| Texas Instruments Incorporated
| TUSB9261 TUSB 3.0 to SATA Bridge
| Marketing part#   Voltage Range   Package-type   Temperature
| TUSB9261PAP   2.97V - 3.465V   64-Pin TQFP   -40 to 105 C
| TUSB9261PVP   2.97V - 3.465V   64-Pin TQFP   -40 to 105 C
[IBIS Ver]   4.0
[File name]   tusb9261.ibs
[File Rev]   1.0
[Date]   12/17/2010
[Source]   Model built from TISPICE simulations at:
   Texas Instruments Incorporated.
   Analog-eLab, HPA
   12500 TI Blvd
   Dallas, TX -75243
   For Support e-mail: elab_scm_ibis@list.ti.com
[Notes]   Rev 1.0: 12/17/2010
   - Model based on tusb1310.ibs v1.1 IBIS model.
   - Model generated from simulations in TISPICED
   - For USB2.0, models are included for HS, FS and LS modes
   - For USB3.0, models are included for SATA1, SATA2 and No-De-Emphasis
   modes
   - USB2 and USB3  models are matched to TISPICE.
   - Added model for DeEmphasis mode
   - Please use [Package Model] for system analysis
   - C_comp although listed in numerical order of value are obtained from varying
   PVT conditions. For PVT conditions for each specific value refer the buffer
   description under respective [Model]. IBIS model user is responsible for using
   appropriate C_comp to simulate for Signal Integrity
   Where for TUSB1310,
   Nom PVT:  Nominal process, Typ Temperature, Typ Voltage
   Slow PVT: Weak process, Max Temperature, Min Voltage
   Fast PVT: Strong process, Min Temperature, Max Voltage
   - ignore warning are related to usb3_WODE, please do not correct this error
   as IBIS parser does not correct IV-VT mismatch with single set of V-T
   waveforms.
   - non-monotonic arnings related to usb2_LS_RC and usb2_LS_R buffers are
   as they are seen in TISPICE simualations
   - [Driver Schedule] is interpreted differently by each system level simulator
   differently, if usual setup with it does not give appropriate results, please
   tie the MAIN and BOOST buffers as per buffer timing description under
   [Driver Schedule] keyword. For example, using HSPICE, refer DE_hspice.sp
   - To test USB2 IBIS models using HSPICE look for spice set up files
   inside the TUSB1310 Correlation report
   - Both PVP and PAP packages have same parasitics
   - Digital models are from standard ASIC SR60 IBIS library for TUSB9261
[Disclaimer] This product is designed as an aid for customers of Texas Instruments.
   No warranties, either expressed or implied, with respect to this third
   party software (if any) or with respect to its fitness for any
   particular purpose is claimed by Texas Instruments or the author. The
   software (if any) is provided solely on an "as is" basis. The entire
   risk as to its quality and performance is with the customer
[Copyright]   (C)Copyright 2010 Texas Instruments Incorporated.
   All rights reserved.
|   TUSB9261 PAP 64-pin TQFP with thermal pad
[Component]   TUSB9261PAP
[Manufacturer]  Texas Instruments Incorporated
[Package]   |65-pin PAP TQFP
|   typ   min   max
R_pkg   0.211135   0.01351   0.24747
L_pkg   2.91049nH   1.34206nH   3.55002nH
C_pkg   0.62782pF   0.45374pF   0.68688pF
[PIN]  Signal_name   Model_name   R_pin   L_pin   C_pin
1   VDD   POWER   0.13086   3.225576nH   0.70225pF
2   PWM0   BC3340DSHYPBFZP18PD  0.23767   3.369912nH   0.67131pF
3   PWM1   BC3340DSHYPBFZP18PD  0.22511   3.211136nH   0.65435pF
4   GRSTZ   IC33SHYPBFZP18PU   0.21557   3.084096nH   0.63183pF
5   UART_RX_GPIO8  BC3340DSHYPBFZP18PU  0.21063   3.003016nH   0.62696pF
6   UART_TX_GPIO9  BC3340DSHYPBFZP18PU  0.20875   2.955072nH   0.62244pF
7   VDD33   POWER   0.10961   2.607272nH   0.64774pF
8   GPIO0   BC3340DSHYPBFZP18PD  0.20588   2.88772nH   0.58903pF
9   GPIO1   BC3340DSHYPBFZP18PD  0.20559   2.88536nH   0.5925pF
10   GPIO2   BC3340DSHYPBFZP18PD  0.20518   2.898064nH   0.61553pF
11   GPIO3   BC3340DSHYPBFZP18PD  0.20774   2.947056nH   0.60753pF
12   VDD   POWER   0.11187   2.699616nH   0.66867pF
13   GPIO4   BC3340DSHYPBFZP18PD  0.21619   3.092752nH   0.64028pF
14   GPIO5   BC3340DSHYPBFZP18PD  0.2259   3.222312nH   0.66752pF
15   GPIO6   BC3340DSHYPBFZP18PD  0.23204   3.320784nH   0.68037pF
16   GPIO7   BC3340DSHYPBFZP18PD  0.24662   3.541544nH   0.62837pF
17   SPI_SCLK   BC3340DSHYPBFZP18PU  0.24747   3.550024nH   0.64185pF
18   SPI_DATA_IN   IC33SHYPBFZP18PU   0.23987   3.395592nH   0.68688pF
19   VDD   POWER   0.12307   2.9634nH   0.71297pF
20   SPI_DATA_OUT   BC3340DSHYPBFZP18PU  0.2236   3.164256nH   0.65587pF
21   SPI_CS0   BC3340DSHYPBFZP18PU  0.22022   3.097736nH   0.6409pF
22   SPI_CS1_GPIO10 BC3340DSHYPBFZP18PU  0.21452   3.013472nH   0.61593pF
23   SPI_CS2_GPIO11 BC3340DSHYPBFZP18PU  0.21142   2.959624nH   0.60709pF
24   VDD33   POWER   0.112   2.631416nH   0.65058pF
25   JTAG_TCK   IC33SHYPBFZP18PD   0.21142   2.94336nH   0.59887pF
26   JTAG_TDI   IC33SHYPBFZP18PU   0.21121   2.957824nH   0.62272pF
27   JTAG_TDO   BC3340DSHYPBFZP18PD  0.21414   3.009856nH   0.61076pF
28   JTAG_TMS   IC33SHYPBFZP18PU   0.21773   3.074424nH   0.62341pF
29   JTAG_TRSTZ   IC33SHYPBFZP18PD   0.22537   3.180992nH   0.65602pF
30   FREQSEL0   IC33SHYPBFZP18PU   0.22999   3.262152nH   0.66926pF
31   FREQSEL1   IC33SHYPBFZP18PU   0.24224   3.418064nH   0.67295pF
32   VDD   POWER   0.09526   3.587624nH   0.70248pF
33   VDD   POWER   0.26179   3.685304nH   0.65998pF
34   VDDA33   POWER   0.23867   3.383512nH   0.67901pF
35   USB_DM   usb2   0.2264   3.226896nH   0.65519pF
36   USB_DP   usb2   0.21671   3.097536nH   0.63419pF
37   NC   NC   0.01351   1.342056nH   0.47338pF
38   USB_R1   NC   0.2087   2.956272nH   0.60989pF
39   USB_R1RTN   NC   0.20571   2.903064nH   0.5999pF
40   VDDA33   POWER   0.2054   2.88348nH   0.59106pF
41   VDD   POWER   0.08086   2.864096nH   0.65481pF
42   USB_SSTX_N   usb3   0.20711   2.186388nH   0.60301pF
43   USB_SSTX_P   usb3   0.21108   2.232552nH   0.61344pF
44   NC   NC   0.21761   3.068664nH   0.62787pF
45   USB_SSRX_N   RXP_N   0.22603   2.386884nH   0.66154pF
46   USB_SSRX_P   RXP_N   0.23763   2.496954nH   0.6838pF
47   VDD   POWER   0.09682   3.705672nH   0.78409pF
48   VDDR33   POWER   0.27024   3.760504nH   0.65113pF
49   VDD   POWER   0.09565   3.189344nH   0.7401pF
50   USB_VBUS   NC   0.24038   3.394712nH   0.67398pF
51   VDD33   POWER   0.12314   2.989664nH   0.71237pF
52   XI   NC   0.22287   3.151136nH   0.64979pF
53   VSSOSC   GND   0.21544   3.046216nH   0.63062pF
54   XO   NC   0.2111   2.974672nH   0.63043pF
55   VDD   POWER   0.11418   2.729152nH   0.6819pF
56   SATA_TX_N   SATA   0.21102   2.19969nH   0.59907pF
57   SATA_TX_P   SATA   0.21296   2.2134nH   0.59744pF
58   NC   NC   0.21605   2.996784nH   0.61426pF
59   SATA_RX_N   RXP_N   0.22106   2.301492nH   0.64313pF
60   SATA_RX_P   RXP_N   0.22882   2.379558nH   0.64598pF
61   VDD   POWER   0.0925   3.52468nH   0.7389pF
62   VDDR33   POWER   0.25481   3.491112nH   0.67158pF
63   VDD   POWER   0.25401   3.523744nH   0.67646pF
64   NC   NC   0.01425   1.544184nH   0.45374pF
65   VSS   GND   0.0001   0.0001nH   0.0001pF|THERMAL PAD
|   TUSB9261 PVP 64-pin TQFP with thermal pad
[Component]   TUSB9261PVP
[Manufacturer]  Texas Instruments Incorporated
[Package]   |65-pin PVP TQFP
|   typ   min   max
R_pkg   0.211135   0.01351   0.24747
L_pkg   2.22301nH   0.82343nH   2.83923nH
C_pkg   0.626679pF   0.45374pF   0.68688pF
[PIN]  Signal_name   Model_name   R_pin   L_pin   C_pin
1   VDD   POWER   0.13086   2.466064nH   0.70225pF
2   PWM0   BC3340DSHYPBFZP18PD  0.23767   2.671448nH   0.67131pF
3   PWM1   BC3340DSHYPBFZP18PD  0.22511   2.515544nH   0.65435pF
4   GRSTZ   IC33SHYPBFZP18PU   0.21557   2.365448nH   0.63183pF
5   UART_RX_GPIO8  BC3340DSHYPBFZP18PU  0.21063   3.003016nH   0.62696pF
6   UART_TX_GPIO9  BC3340DSHYPBFZP18PU  0.20875   2.278152nH   0.62244pF
7   VDD33   POWER   0.10961   1.910424nH   0.64774pF
8   GPIO0   BC3340DSHYPBFZP18PD  0.20588   2.142112nH   0.58903pF
9   GPIO1   BC3340DSHYPBFZP18PD  0.20559   2.150664nH   0.5925pF
10   GPIO2   BC3340DSHYPBFZP18PD  0.20518   2.180696nH   0.61553pF
11   GPIO3   BC3340DSHYPBFZP18PD  0.20774   2.223272nH   0.60753pF
12   VDD   POWER   0.11187   1.988264nH   0.66867pF
13   GPIO4   BC3340DSHYPBFZP18PD  0.21619   2.37416nH   0.64028pF
14   GPIO5   BC3340DSHYPBFZP18PD  0.2259   2.526576nH   0.66752pF
15   GPIO6   BC3340DSHYPBFZP18PD  0.23204   2.624064nH   0.68037pF
16   GPIO7   BC3340DSHYPBFZP18PD  0.24662   2.837376nH   0.62837pF
17   SPI_SCLK   BC3340DSHYPBFZP18PU  0.24747   2.839232nH   0.64185pF
18   SPI_DATA_IN   IC33SHYPBFZP18PU   0.23987   2.697288nH   0.68688pF
19   VDD   POWER   0.12307   2.274824nH   0.71297pF
20   SPI_DATA_OUT   BC3340DSHYPBFZP18PU  0.2236   2.445128nH   0.65587pF
21   SPI_CS0   BC3340DSHYPBFZP18PU  0.22022   2.372392nH   0.6409pF
22   SPI_CS1_GPIO10 BC3340DSHYPBFZP18PU  0.21452   2.289296nH   0.61593pF
23   SPI_CS2_GPIO11 BC3340DSHYPBFZP18PU  0.21142   2.2416nH   0.60709pF
24   VDD33   POWER   0.112   1.90852nH   0.65058pF
25   JTAG_TCK   IC33SHYPBFZP18PD   0.21142   2.208344nH   0.59887pF
26   JTAG_TDI   IC33SHYPBFZP18PU   0.21121   2.239896nH   0.62272pF
27   JTAG_TDO   BC3340DSHYPBFZP18PD  0.21414   2.285672nH   0.61076pF
28   JTAG_TMS   IC33SHYPBFZP18PU   0.21773   2.348848nH   0.62341pF
29   JTAG_TRSTZ   IC33SHYPBFZP18PD   0.22537   2.46208nH   0.65602pF
30   FREQSEL0   IC33SHYPBFZP18PU   0.22999   2.566816nH   0.66926pF
31   FREQSEL1   IC33SHYPBFZP18PU   0.24224   2.721184nH   0.67295pF
32   VDD   POWER   0.09526   2.467272nH   0.70248pF
33   VDD   POWER   0.26179   2.976512nH   0.65998pF
34   VDDA33   POWER   0.23867   2.685288nH   0.67901pF
35   USB_DM   usb2   0.2264   2.531224nH   0.65519pF
36   USB_DP   usb2   0.21671   2.378968nH   0.63419pF
37   NC   NC   0.01351   0.823432nH   0.47338pF
38   USB_R1   NC   0.2087   2.232496nH   0.60989pF
39   USB_R1RTN   NC   0.20571   2.18544nH   0.5999pF
40   VDDA33   POWER   0.2054   2.137712nH   0.59106pF
41   VDD   POWER   0.08086   2.121728nH   0.65481pF
42   USB_SSTX_N   usb3   0.20711   1.648002nH   0.60301pF
43   USB_SSTX_P   usb3   0.21108   1.689534nH   0.61344pF
44   NC   NC   0.21761   2.343088nH   0.62787pF
45   USB_SSRX_N   RXP_N   0.22603   1.975452nH   0.66154pF
46   USB_SSRX_P   RXP_N   0.23763   1.975452nH   0.6838pF
47   VDD   POWER   0.09682   3.020784nH   0.78409pF
48   VDDR33   POWER   0.27024   3.058096nH   0.65113pF
49   VDD   POWER   0.09565   2.215056nH   0.7401pF
50   USB_VBUS   NC   0.24038   2.696408nH   0.67398pF
51   VDD33   POWER   0.12314   2.297232nH   0.71237pF
52   XI   NC   0.22287   2.432248nH   0.64979pF
53   VSSOSC   GND   0.21544   2.321352nH   0.63062pF
54   XO   NC   0.2111   2.251696nH   0.63043pF
55   VDD   POWER   0.11418   2.015832nH   0.6819pF
56   SATA_TX_N   SATA   0.21102   1.640724nH   0.59907pF
57   SATA_TX_P   SATA   0.21296   1.662558nH   0.59744pF
58   NC   NC   0.21605   2.279256nH   0.61426pF
59   SATA_RX_N   RXP_N   0.22106   1.758834nH   0.64313pF
60   SATA_RX_P   RXP_N   0.22882   1.835676nH   0.64598pF
61   VDD   POWER   0.0925   2.631208nH   0.7389pF
62   VDDR33   POWER   0.25481   2.795136nH   0.67158pF
63   VDD   POWER   0.25401   2.826544nH   0.67646pF
64   NC   NC   0.01425   0.983936nH   0.45374pF
65   VSS   GND   0.0001   0.0001nH   0.0001pF|THERMAL PAD
[Diff_pin]   inv_pin   vdiff   tdelay_typ   tdelay_min   tdelay_max
36   35   880mV   NA NA NA|USB_DP/DM
43   42   NA   NA NA NA| USB_SSTXP/N
46   45   2200mV   NA NA NA| USB_SSRXP/N
57   56   NA   NA NA NA| SATA_TXP/N
60   59   2200mV   NA NA NA| SATA_RXP/N
[Pin Mapping] pulldown_ref pullup_ref gnd_clamp_ref power_clamp_ref |ext_ref
1   NC   VDD11BUS
2   VSSBUS   VDD33BUS   VSSBUS   VDD33BUS
3   VSSBUS   VDD33BUS   VSSBUS   VDD33BUS
4   NC   NC   VSSBUS   VDD33BUS
5   VSSBUS   VDD33BUS   VSSBUS   VDD33BUS
6   VSSBUS   VDD33BUS   VSSBUS   VDD33BUS
7   NC   VDD33BUS
8   VSSBUS   VDD33BUS   VSSBUS   VDD33BUS
9   VSSBUS   VDD33BUS   VSSBUS   VDD33BUS
10   VSSBUS   VDD33BUS   VSSBUS   VDD33BUS
11   VSSBUS   VDD33BUS   VSSBUS   VDD33BUS
12   NC   VDD11BUS
13   VSSBUS   VDD33BUS   VSSBUS   VDD33BUS
14   VSSBUS   VDD33BUS   VSSBUS   VDD33BUS
15   VSSBUS   VDD33BUS   VSSBUS   VDD33BUS
16   VSSBUS   VDD33BUS   VSSBUS   VDD33BUS
17   VSSBUS   VDD33BUS   VSSBUS   VDD33BUS
18   NC   NC   VSSBUS   VDD33BUS
19   NC   VDD11BUS
20   VSSBUS   VDD33BUS   VSSBUS   VDD33BUS
21   VSSBUS   VDD33BUS   VSSBUS   VDD33BUS
22   VSSBUS   VDD33BUS   VSSBUS   VDD33BUS
23   VSSBUS   VDD33BUS   VSSBUS   VDD33BUS
24   NC   VDD33BUS
25   NC   NC   VSSBUS   VDD33BUS
26   NC   NC   VSSBUS   VDD33BUS
27   VSSBUS   VDD33BUS   VSSBUS   VDD33BUS
28   NC   NC   VSSBUS   VDD33BUS
29   NC   NC   VSSBUS   VDD33BUS
30   NC   NC   VSSBUS   VDD33BUS
31   NC   NC   VSSBUS   VDD33BUS
32   NC   VDD11BUS
33   NC   VDD11BUS
34   NC   VDDA33BUS
35   VSSBUS   VDD33BUS   VSSBUS   VDD33BUS
36   VSSBUS   VDD33BUS   VSSBUS   VDD33BUS
37   NC   NC
38   NC   NC
39   NC   NC
40   NC   VDDA33
41   NC   VDD11BUS
42   VSSBUS   VDD11BUS   VSSBUS   VDD11BUS
43   VSSBUS   VDD11BUS   VSSBUS   VDD11BUS
44   NC   NC
45   NC   NC   VSSBUS   VDD11BUS
46   NC   NC   VSSBUS   VDD11BUS
47   NC   VDD11BUS
48   NC   VDDR33BUS
49   NC   VDD11BUS
50   NC   NC
51   NC   VDD33BUS
52   NC   NC
53   VSSBUS   NC
54   NC   NC
55   NC   VDD11BUS
56   VSSBUS   VDD11BUS   VSSBUS   VDD11BUS
57   VSSBUS   VDD11BUS   VSSBUS   VDD11BUS
58   NC   NC
59   NC   NC   VSSBUS   VDD11BUS
60   NC   NC   VSSBUS   VDD11BUS
61   NC   VDD11BUS
62   NC   VDDR33BUS
63   NC   VDD11BUS
64   NC   NC
65   VSSBUS   NC
[Model Selector] usb2
usb2_HS_R   USB 2.0 High Speed mode, for DP/DM pin 240MHz
usb2_HS_RC   USB 2.0 High Speed mode, for DP/DM pin 240MHz, with Cfixture
usb2_FS_R   USB 2.0 Fast Speed mode, for DP/DM pin 6MHz
usb2_FS_RC   USB 2.0 Fast Speed mode, for DP/DM pin 6MHz, with Cfixture
usb2_LS_RC   USB 2.0 Low  Speed mode, for DP/DM pin 750kHz, with Cfixture
usb2_LS_R   USB 2.0 Low  Speed mode, for DP/DM pin 750kHz
[Model Selector] usb3
usb3_DE   USB 3.0 De-Emphasis mode, best at 1.25GHz
usb3_WODE   USB 3.0 No De-Emphasis mode, for SSTXP/N 2.5GHz
usb3_SATA1   USB 3.0 SATA1 mode, for SSTXP/N 750MHz
usb3_SATA2   USB 3.0 SATA2 mode, for SSTXP/N 1.5GHz
[Model Selector] SATA
usb3_SATA1   USB 3.0 SATA1 mode, for SSTXP/N 750MHz
usb3_SATA2   USB 3.0 SATA2 mode, for SSTXP/N 1.5GHz
[Model Selector] BC3340DSHYPBFZP18
HYPBFZP18_PI_5P_3P3 BUFFER WITHOUT PULLUP/PULLDOWN & 5% VDDS TOLERANCE
HYPBFZP18_PI_10P_3P3 BUFFER WITHOUT PULLUP/PULLDOWN & 10% VDDS TOLERANCE
[Model Selector] BC3340DSHYPBFZP18PU
FZP18_PU_PI_5P_3P3 BUFFER WITH WEAK PULLUP & 5% VDDS TOLERANCE
FZP18_PU_PI_10P_3P3 BUFFER WITH WEAK PULLUP & 10% VDDS TOLERANCE
[Model Selector] BC3340DSHYPBFZP18PD
FZP18_PD_PI_5P_3P3 BUFFER WITH WEAK PULLDOWN & 5% VDDS TOLERANCE
FZP18_PD_PI_10P_3P3 BUFFER WITH WEAK PULLDOWN & 10% VDDS TOLERANCE
[Model Selector] IC33SHYPBFZP18
C33SHYPBFZP18_10P BUFFER WITHOUT PULLUP/PULLDOWN & 10% VDDS TOLERANCE
C33SHYPBFZP18_5P  BUFFER WITHOUT PULLUP/PULLDOWN & 5% VDDS TOLERANCE
[Model Selector] IC33SHYPBFZP18PD
YPBFZP18_PD_5P BUFFER with WEAK PULLDOWN & 5% VDDS TOLERANCE
YPBFZP18_PD_10P BUFFER with WEAK PULLDOWN & 5% VDDS TOLERANCE
[Model Selector] IC33SHYPBFZP18PU
PBFZP18_PU_5P BUFFER with WEAK PULLUP & 5% VDDS TOLERANCE
PBFZP18_PU_10P BUFFER with WEAK PULLUP & 10% VDDS TOLERANCE
|USB 3.0 De-Emphasis mode, for SSTXP/SSTXN pins 2.5Gbps(1.25GHz to De-Emphasis)
[Model]   usb3_DE
Model_type   Output
Vmeas = 1.1
Vref = 1.1
Rref = 50
|   typ   min   max
|   (TYP PVT)   (Fast PVT) (Slow PVT)
C_comp   0pF   0pF   0pF
[Driver Schedule]
| Model_name   Rise_on_dly Rise_off_dly Fall_on_dly Fall_off_dly
usb3_de_MAIN   0.0nS   0.4ns   0   0.4ns
usb3_de_BOOST   0.0nS   0.2nS   0   0.2nS
[Voltage Range]   1.1   0.99   1.155
[Temperature Range]   27   105   -40
[Pullup Reference]   1.1   0.99   1.155
[Pulldown Reference]   0   0   0
[Power Clamp Reference]   1.1   0.99   1.155
[GND Clamp Reference]   0   0   0
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[Ramp]
R_load = 50
|   typ   min   max
dV/dt_r   0.972315/1.549e-011   0.988218/1.8606e-011   0.957162/1.40763e-011
dV/dt_f   0.972312/7.7916e-012   0.988183/1.21282e-011  0.957081/6.00194e-012
| Models and submodels in the file (25): RXP_N (Input), usb2_FS_R (I/O), usb2_FS_RC (I/O), usb2_HS_R (I/O), usb2_HS_RC (I/O), usb2_LS_R (I/O), usb2_LS_RC (I/O), usb3_WODE (Output), usb3_SATA1 (Output), usb3_SATA2 (Output), usb3_DE (Output), usb3_de_MAIN (Output), usb3_de_BOOST (Open_drain), HYPBFZP18_PI_5P_3P3 (I/O), HYPBFZP18_PI_10P_3P3 (I/O), FZP18_PU_PI_5P_3P3 (I/O), FZP18_PU_PI_10P_3P3 (I/O), FZP18_PD_PI_5P_3P3 (I/O), FZP18_PD_PI_10P_3P3 (I/O), YPBFZP18_PD_10P (Input), PBFZP18_PU_10P (Input), C33SHYPBFZP18_10P (Input), YPBFZP18_PD_5P (Input), PBFZP18_PU_5P (Input), C33SHYPBFZP18_5P (Input)
